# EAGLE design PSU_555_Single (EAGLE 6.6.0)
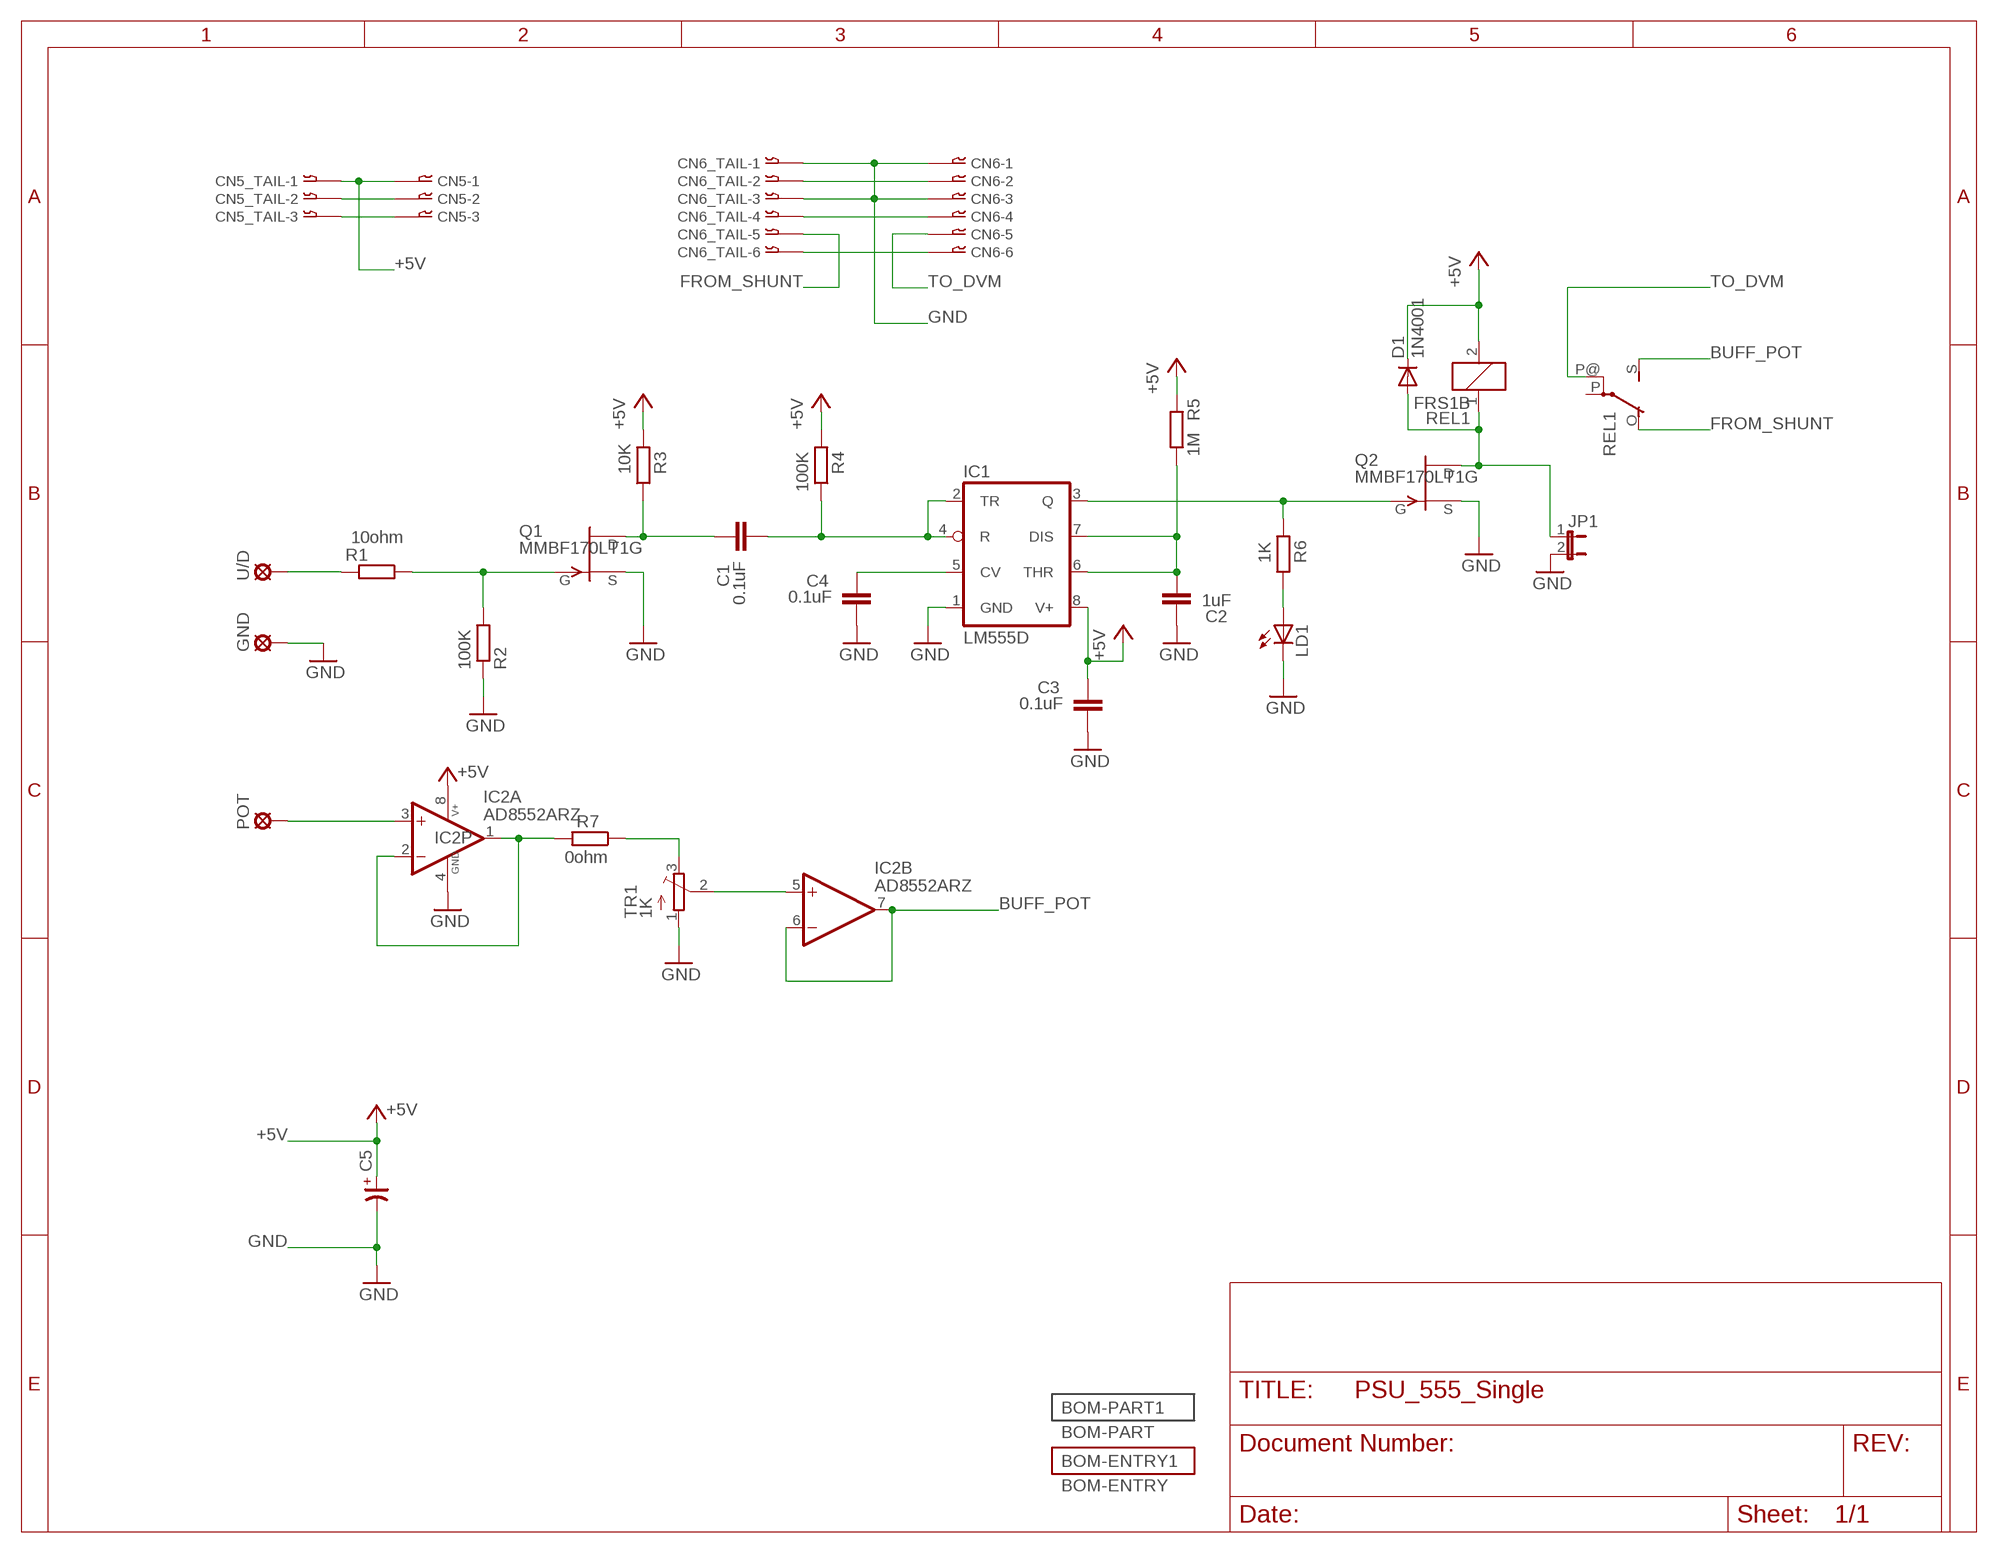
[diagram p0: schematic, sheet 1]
BOM-PART1 (BOM-PART): BOM: INCLUDE; QTY: 1

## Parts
C1  0.1uF  C-EUC0805  [C0805]
C2  1uF  C-EUC0805  [C0805]
C3  0.1uF  C-EUC0805  [C0805]
C4  0.1uF  C-EUC0805  [C0805]
C5  CP-SV-A  [SV-A]
CN5  03-JST-B3B-XH-A  [B3B-XH]
CN5_TAIL  03-JST-B3B-XH-A  [B3B-XH]
CN6  06-JST-B6B-XH-A  [B6B-XH]
CN6_TAIL  06-JST-B6B-XH-A  [B6B-XH]
D1  1N4001  ES2D  [SMB]
GND  SE11  [SE11]
IC1  LM555D  [SO08]
IC2  AD8552ARZ  LM358D  [SO08]
JP1  JP1E  [JP1]
LD1  LEDSML0805  [SML0805]
POT  SE11  [SE11]
Q1  MMBF170LT1G  [SOT23]
Q2  MMBF170LT1G  [SOT23]
R1  10ohm  R-EU_R0805  [R0805]
R2  100K  R-EU_R0805  [R0805]
R3  10K  R-EU_R0805  [R0805]
R4  100K  R-EU_R0805  [R0805]
R5  1M  R-EU_R0805  [R0805]
R6  1K  R-EU_R0805  [R0805]
R7  0ohm  R-EU_R0805  [R0805]
REL1  FRS1B  [FRS1B]
TR1  1K  TRIM_EU-3223W  [3223W]
U/D  SE11  [SE11]

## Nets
+5V: C3.1 C5.+ CN5.P$1 CN5_TAIL.P$1 D1.C IC1.8(V+) IC2.8(P:V+) R3.2 R4.2 R5.2 REL1.2
BUFF_POT: IC2.6(B:-IN) IC2.7(B:OUT) REL1.S(2:S)
FROM_SHUNT: CN6_TAIL.P$5 REL1.O(2:O)
GND: C2.1 C3.2 C4.2 C5.- CN6.P$1 CN6.P$3 CN6_TAIL.P$1 CN6_TAIL.P$3 GND.MP IC1.1(GND) IC2.4(P:GND) JP1.2 LD1.C Q1.2(S) Q2.2(S) R2.1 TR1.1(A)
N$1: LD1.A R6.1
N$2: IC2.1(A:OUT) IC2.2(A:-IN) R7.2
N$3: Q1.1(G) R1.1 R2.2
N$4: C1.1 Q1.3(D) R3.1
N$5: R1.2 U/D.MP
N$6: C1.2 IC1.2(TR) IC1.4(R) R4.1
N$7: D1.A JP1.1 Q2.3(D) REL1.1
N$8: IC2.5(B:+IN) TR1.2(S)
N$9: IC2.3(A:+IN) POT.MP
N$10: IC1.3(Q) Q2.1(G) R6.2
N$11: C2.2 IC1.6(THR) IC1.7(DIS) R5.1
N$12: CN5.P$2 CN5_TAIL.P$2
N$15: R7.1 TR1.3(E)
N$16: C4.1 IC1.5(CV)
N$17: CN5.P$3 CN5_TAIL.P$3
N$25: CN6.P$2 CN6_TAIL.P$2
N$27: CN6.P$4 CN6_TAIL.P$4
N$28: CN6.P$6 CN6_TAIL.P$6
TO_DVM: CN6.P$5 REL1.P@(2:P)
Unconnected: REL1.P(2:P)

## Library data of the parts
C1-C4 = rcl:C-EU: CAPACITOR, European symbol
C5 = cap-master:CP-: POLARIZED CAP
CN5 CN5_TAIL = con-jst-xh:03-JST: JST CONNECTOR
CN6 CN6_TAIL = con-jst-xh:06-JST: JST CONNECTOR
D1 = diode:ES2D: DIODE
GND POT U/D = solpad:SE11: SOLDER PAD
IC1 = linear:*555: TIMER
IC2 = op-amp:LM358: OP-AMP - Dual
JP1 = jumper:JP1E: JUMPER
LD1 = led:LED: LED
Q1 Q2 = transistor-fet:MMBF170LT1G
R1-R7 = rcl:R-EU_: RESISTOR, European symbol
REL1 = relay:FRS1B: RELAY 1 x switch, same as V23101-D6-A201, Siemens; OC_FARNELL: unknown; OC_NEWARK: unknown; PARTNO: RS 476-731
TR1 = pot:TRIM_EU-: POTENTIOMETER

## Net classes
1 vcc: width 0.254 mm
2 gnd: width 0.254 mm, drill 0.61 mm, clearance 0.254 mm
3 usbvcc: width 0.254 mm, drill 0.61 mm, clearance 0.254 mm
4 aref: width 0.254 mm, drill 0.61 mm, clearance 0.254 mm

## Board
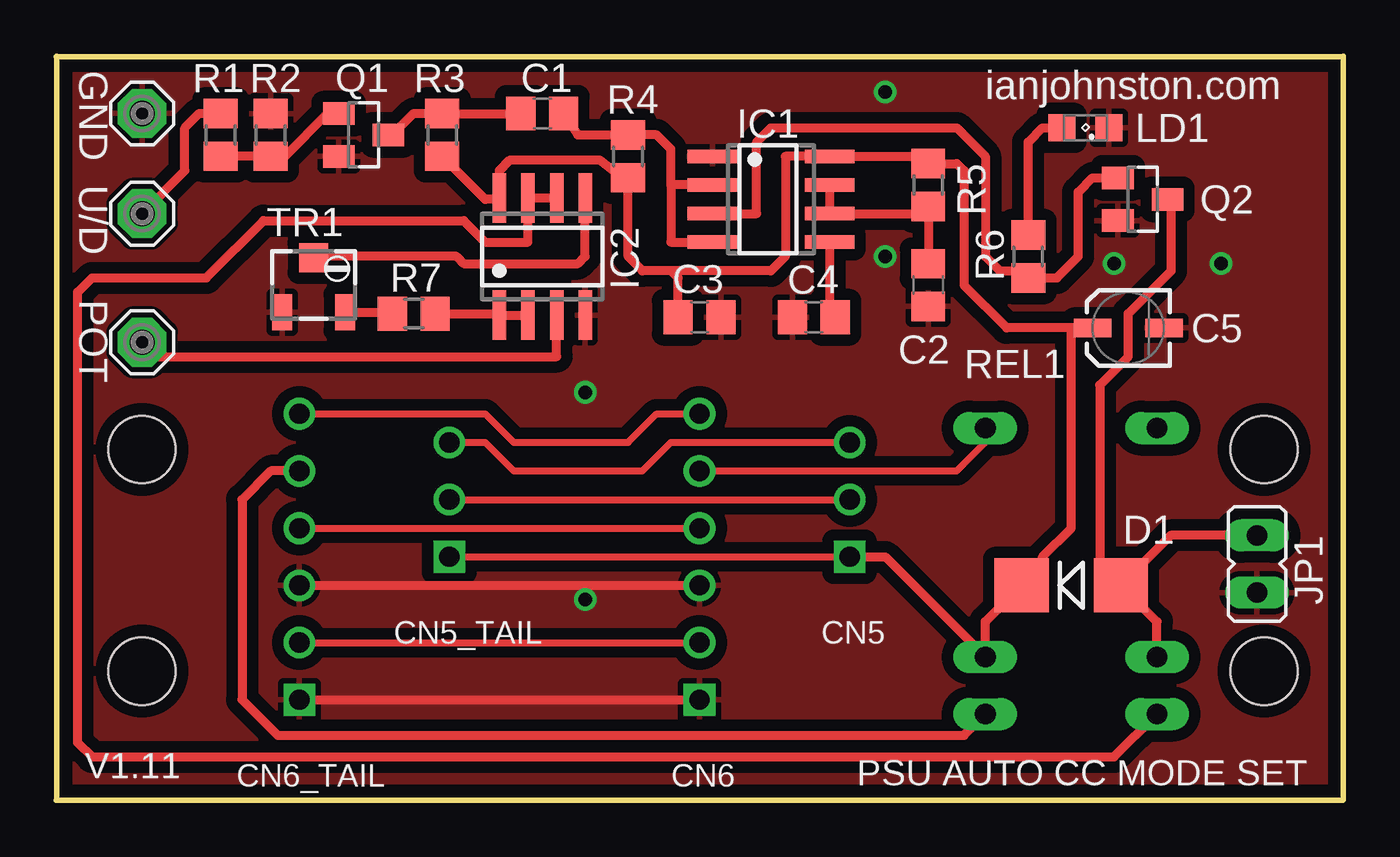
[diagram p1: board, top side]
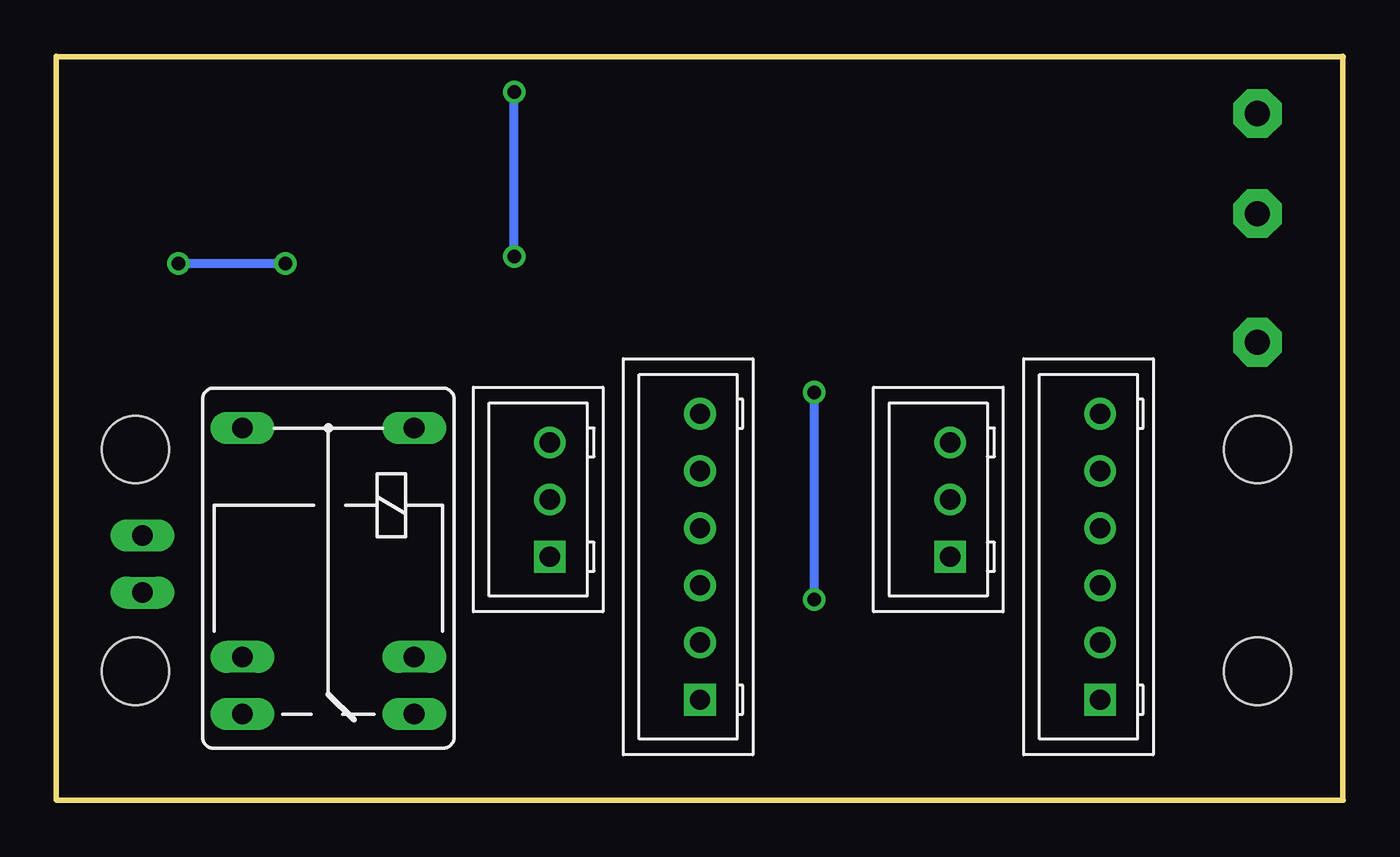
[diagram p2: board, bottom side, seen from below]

Size 57.17 x 33.04 mm. Coordinates in mm from the lower left corner, seen from the top.
Outline: 57.15,0 0,0
Outline: 0.02,33.04 0.02,0.02
Outline: 57.17,33.04 57.17,0.02
Outline: 57.15,33.02 0,33.02
Copper layers (1*16): Top 0.035mm / dielectric 1.5mm / Bottom 0.035mm
Design rules "default *": minimum track width 10mil, minimum drill 24mil, track to track 20mil, track to pad 20mil, pad to pad 20mil, via to via 20mil, smd to smd 20mil, copper to edge 22mil, drill to drill 8mil, minimum pad ring 10mil, minimum via ring 8mil, stop-mask expansion 4mil, vias tented up to drill 0mil, thermal gap 10mil
Holes 3 mm at 3.81,15.58 3.81,5.74 53.66,5.74 53.66,15.58

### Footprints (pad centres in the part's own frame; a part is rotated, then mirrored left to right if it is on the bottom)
C0805 = smd 1.3 x 1.5: 1 -0.95,0; 2 0.95,0
SV-A = smd 1.676 x 0.813: + -1.587,0; - 1.587,0
B3B-XH = drill 0.9 square: P$1 -2.54,0 | drill 0.9: P$2 0,0; P$3 2.54,0
B6B-XH = drill 0.9 square: P$1 -6.35,0 | drill 0.9: P$2 -3.81,0; P$3 -1.27,0; P$4 1.27,0; P$5 3.81,0; P$6 6.35,0
SMB = smd 2.4 x 2.4: A 2.2,0; C -2.2,0
SE11 = drill 1.118 pad 2.159 octagon: MP 0,0
SO08 = smd 0.6 x 2.2: 1 -1.905,-2.6; 2 -0.635,-2.6; 3 0.635,-2.6; 4 1.905,-2.6; 5 1.905,2.6; 6 0.635,2.6; 7 -0.635,2.6; 8 -1.905,2.6
JP1 = drill 0.914 long: 1 0,-1.27; 2 0,1.27
SML0805 = smd 1.2 x 1.2: A 1.05,0; C -1.05,0
SOT23 = smd 1 x 1.4: 1 -0.95,-1.1; 2 0.95,-1.1; 3 0,1.1
R0805 = smd 1.3 x 1.5: 1 -0.95,0; 2 0.95,0
FRS1B = drill 0.914 long: 1 0,3.81; 2 0,-3.81; O -2.54,-3.81; P 10.16,3.81; P@ 10.16,-3.81; S -2.54,3.81
3223W = smd 0.9 x 1.6: 1 -1.4,-1.215; 3 1.4,-1.215 | smd 1.3 x 1.3: 2 0,1.215

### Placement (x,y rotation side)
C1  21.59,30.5 0 top
C2  38.73,22.88 90 top
C3  28.57,21.45 0 top
C4  33.66,21.45 180 top
C5  47.62,20.98 0 top
CN5  35.24,13.36 90 bottom
CN5_TAIL  17.46,13.36 90 bottom
CN6  28.57,10.82 90 bottom
CN6_TAIL  10.79,10.82 90 bottom
D1  45.09,9.55 0 top
GND  3.81,30.5 0 top
IC1  31.75,26.69 270 top
IC2  21.59,24.15 0 top
JP1  53.34,10.5 180 top
LD1  45.72,29.87 180 top
POT  3.81,20.34 0 top
Q1  13.65,29.55 270 top
Q2  48.26,26.69 270 top
R1  7.3,29.55 90 top
R2  9.53,29.55 270 top
R3  17.14,29.55 270 top
R4  25.4,28.6 270 top
R5  38.73,27.33 90 top
R6  43.18,24.15 270 top
R7  15.88,21.61 0 top
REL1  45.09,6.37 90 bottom
TR1  11.43,22.88 0 top
U/D  3.81,26.06 0 top

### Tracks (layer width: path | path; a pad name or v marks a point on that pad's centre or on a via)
+5V
  Top 0.254: 19.68,26.69 IC2.8
  Top 0.305: CN5_TAIL.P$1 CN5.P$1
  Top 0.406: 19.68,26.69 19.05,26.69 18.41,27.33 18.1,27.64 R3.2 | IC2.8 19.68,27.96 20.16,28.44 24.13,28.44 24.77,27.96 25.09,27.96 R4.2 25.4,24.15 26.04,23.52 27.3,23.52 | C5.+ 45.09,20.98 | 45.09,20.98 42.23,20.98 40.32,22.88 40.32,27.96 40.01,28.28 R5.2 38.73,28.6 IC1.8 32.38,28.6 32.38,24.15 31.75,23.52 27.3,23.52 | C3.1 27.62,23.2 27.3,23.52 | 45.09,20.98 45.09,12.09 43.81,10.82 43.81,10.18 43.18,9.55 D1.C 41.27,7.94 REL1.2 36.83,10.82 CN5.P$1
BUFF_POT
  Top 0.406: IC2.6 IC2.7 20.95,24.79 19.05,24.79 18.1,25.74 9.21,25.74 6.67,23.2 1.59,23.2 0.95,22.57 0.95,2.56 1.59,1.93 46.99,1.93 REL1.S
FROM_SHUNT
  Top 0.406: CN6_TAIL.P$5 9.53,14.63 8.26,13.36 8.26,4.47 9.84,2.88 40.32,2.88 REL1.O
GND  (via drill 0.6)
  Top 0.254: IC2.4 23.5,21.61 23.43,21.62
  Top 0.406: CN6_TAIL.P$1 CN6.P$1 | CN6_TAIL.P$3 CN6.P$3
  Bottom 0.406: v36.83,24.15 v36.83,31.46 | v46.99,23.83 v51.75,23.83 | v23.5,8.91 v23.5,18.12
  pour Top (isolate 0.508): 0.25,32.83 0.25,0.25 56.9,0.25 56.9,32.83
N$1
  Top 0.406: R6.1 43.18,29.23 43.81,29.87 LD1.A
N$2
  Top 0.406: IC2.2 IC2.1 19.62,21.61 R7.2
N$3
  Top 0.406: R1.1 R2.2 10.16,28.6 12.06,30.5 Q1.1
N$4
  Top 0.406: 20.32,30.82 C1.1 R3.1 | 17.14,30.97 R3.1 | Q1.3 14.92,29.55 15.88,30.5 R3.1
N$5
  Top 0.406: U/D.MP 5.71,27.96 5.71,29.87 6.35,30.5 R1.2
N$6
  Top 0.406: IC1.2 27.3,27.33 | 27.3,27.33 27.3,24.79 IC1.4 | C1.2 23.18,29.55 R4.1 26.67,29.55 27.3,28.91 27.3,27.33
N$7
  Top 0.406: REL1.1 48.9,7.94 D1.A | D1.A 46.35,10.48 46.35,18.44 47.62,19.71 47.62,21.61 49.53,23.52 49.53,26.52 Q2.3 | JP1.1 49.51,11.77 D1.A
N$8
  Top 0.406: IC2.5 23.5,24.15 23.18,23.83 18.1,23.83 17.78,24.15 11.43,24.15 TR1.2
N$9
  Top 0.406: POT.MP 3.81,19.71 22.23,19.71 IC2.3
N$10
  Top 0.406: IC1.3 31.11,26.06 31.11,29.23 31.75,29.87 40.01,29.87 41.27,28.6 41.27,24.15 41.91,23.52 42.87,23.52 R6.2 44.45,23.2 45.4,24.15 45.4,27.01 46.04,27.64 Q2.1
N$11
  Top 0.406: IC1.7 IC1.6 38.41,26.06 R5.1 C2.2
N$12
  Top 0.305: CN5_TAIL.P$2 CN5.P$2
N$15
  Top 0.406: TR1.3 14.93,21.67 R7.1
N$16
  Top 0.406: IC1.5 34.35,21.71 C4.1
N$17
  Top 0.305: CN5_TAIL.P$3 19.05,15.9 20.32,14.63 26.04,14.63 27.3,15.9 CN5.P$3
N$25
  Top 0.305: CN6_TAIL.P$2 CN6.P$2
N$27
  Top 0.305: CN6_TAIL.P$4 CN6.P$4
N$28
  Top 0.305: CN6_TAIL.P$6 19.05,17.17 20.32,15.9 25.4,15.9 26.67,17.17 CN6.P$6
TO_DVM
  Top 0.305: CN6.P$5 40.01,14.63 41.27,15.9 REL1.P@

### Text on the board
tPlace: ianjohnston.com | V1.11 | PSU AUTO CC MODE SET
